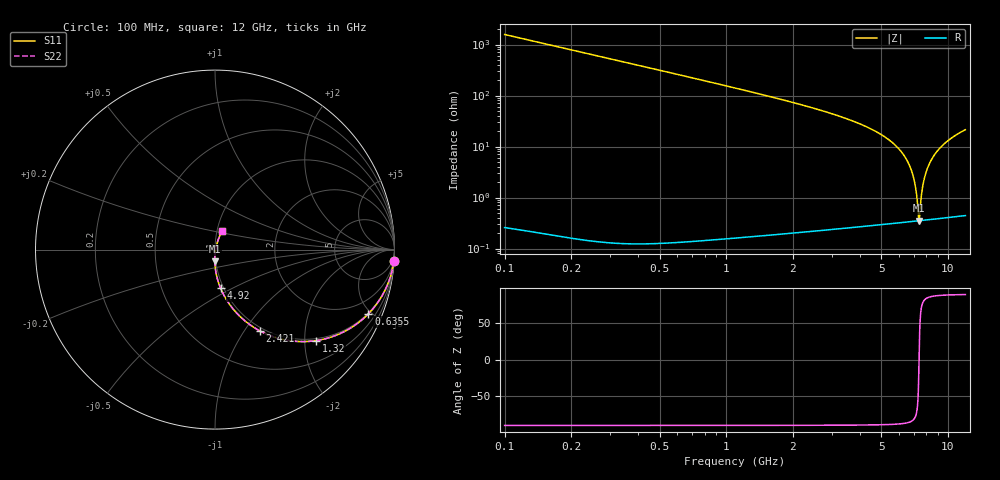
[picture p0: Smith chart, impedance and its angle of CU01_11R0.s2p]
! S-parameter model data by Modelithics Inc. support@modelithics.com 813-866-6335 Tampa FL USA
! S-Parameter data specifications:
! Substrate: 20-mil Rogers, substrate thickness, H=0.508mm, Dielectric constant, Er=3.75
! PCB Mounting Pad Footprint: Pad width, PadW=0.35mm , Pad length, PadL=0.30mm , Pad gap, PadG (edge-to-edge)=0.25mm , Reference planes=0.85mm apart
! Created Tue May  8 14:01:25 2018
# hz S ma R 50
! 2 Port Network Data from SP1.SP block
! freq  magS11  angS11  magS21  angS21  magS12  angS12  magS22  angS22
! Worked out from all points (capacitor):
!   801 points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, 100 MHz to 12 GHz, reference 50 ohm
!   read as one part in series: C = 1.01 pF near 159.5 MHz
!   lowest |Z| = 351 mohm at 7.418 GHz (marker M1)
!   series resonance near 7.414 GHz, so ESL is about 460 pH
!   S11 on the Smith chart (normalised r, x): 100 MHz: 1, -31; 635.5 MHz: 0.95, -4.80; 1.32 GHz: 0.95, -2.27; 2.421 GHz: 0.95, -1.17; 4.92 GHz: 0.97, -0.44; 12 GHz: 1.06, +0.22
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1e8  0.998 -3.7  0.0634 86.3  0.0634 86.3  0.998 -3.7
3.23125e8  0.9795 -11.9  0.2013 78.0  0.2013 78.0  0.9795 -11.9
6.355e8  0.9265 -22.7  0.3759 67.2  0.3759 67.2  0.9265 -22.7
1.31975e9  0.7588 -41.9  0.6501 48.0  0.6501 48.0  0.7588 -41.9
2.09325e9  0.5788 -56.6  0.8137 33.2  0.8137 33.2  0.5788 -56.6
2.4205e9  0.5157 -61.2  0.8549 28.6  0.8549 28.6  0.5157 -61.2
4.071625e9  0.2928 -76.6  0.9536 12.9  0.9536 12.9  0.2928 -76.6
4.9195e9  0.2177 -81.7  0.9731 7.5  0.9731 7.5  0.2177 -81.7
6.05e9  0.1396 -86.9  0.987 1.8  0.987 1.8  0.1396 -86.9
7.4185e9  0.0657 -90.8  0.9943 -3.8  0.9943 -3.8  0.0657 -90.8
8.04325e9  0.03689 -90.5  0.9956 -6.1  0.9956 -6.1  0.03689 -90.5
8.534125e9  0.01602 -84.5  0.9961 -7.8  0.9961 -7.8  0.01602 -84.5
8.682875e9  0.01013 -76.8  0.9961 -8.3  0.9961 -8.3  0.01013 -76.8
8.861375e9  0.004325 -38.8  0.9961 -8.9  0.9961 -8.9  0.004325 -38.8
8.920875e9  0.00377 -5.5  0.9961 -9.1  0.9961 -9.1  0.00377 -5.5
8.980375e9  0.004591 25.4  0.9961 -9.3  0.9961 -9.3  0.004591 25.4
9.17375e9  0.01092 59.6  0.996 -10.0  0.996 -10.0  0.01092 59.6
9.35225e9  0.01757 66.8  0.9959 -10.5  0.9959 -10.5  0.01757 66.8
9.634875e9  0.0281 70.6  0.9956 -11.4  0.9956 -11.4  0.0281 70.6
1.002162e10  0.04221 72.0  0.995 -12.6  0.995 -12.6  0.04221 72.0
1.085462e10  0.0712 71.5  0.9932 -15.2  0.9932 -15.2  0.0712 71.5
1.2e10  0.1084 69.2  0.9896 -18.5  0.9896 -18.5  0.1084 69.2
